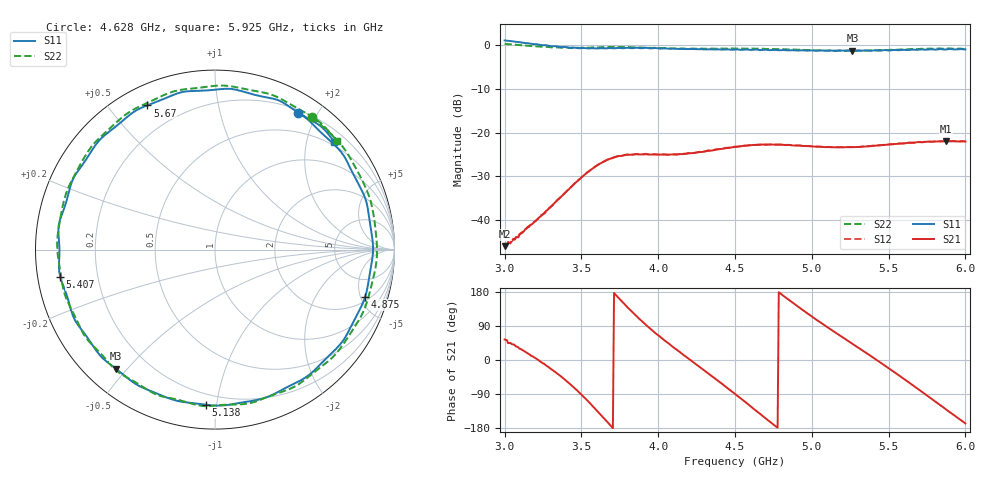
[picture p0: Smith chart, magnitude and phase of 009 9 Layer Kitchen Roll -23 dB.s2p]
!  04/11/2025  15:33:10
! Ref Plane: 0.000 mm
# MHZ S MA R  50
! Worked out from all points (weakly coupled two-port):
!   401 points, 3 GHz to 6 GHz, reference 50 ohm
!   highest |S21| = -22.00 dB at 5.872 GHz (marker M1); lowest = -46.0 dB at 3 GHz (marker M2)
!   lowest |S11| = -1.3 dB at 5.265 GHz (marker M3), VSWR 13.60, Z = 4.48 - j23.3 ohm
!   |S11| at or under -10 dB: nowhere
!   |S22| runs from -1.3 to 0.3 dB; largest |S21 - S12| = 0.0023
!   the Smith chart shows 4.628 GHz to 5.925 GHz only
!   S11 on the Smith chart (normalised r, x): 4.628 GHz: 0.24, +1.75; 4.875 GHz: 2.40, -5.49; 5.138 GHz: 0.14, -0.93; 5.407 GHz: 0.07, -0.09; 5.67 GHz: 0.08, +0.63; 5.925 GHz: 0.42, +2.54
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3000  1.134 -115.5  0.004996 54.1  0.004991 56.0  1.038 -119.1
3270  0.9997 176.6  0.01269 -14.1  0.01247 -11.4  0.9583 173.6
3390  0.9559 138.9  0.02013 -51.0  0.02016 -50.2  0.9414 135.3
3502.5  0.9284 96.3  0.03079 -92.3  0.0307 -91.6  0.9356 92.6
3607.5  0.9192 51.4  0.04263 -136.3  0.04271 -135.6  0.9427 48.3
3735  0.9306 -5.7  0.05337 166.9  0.05364 168.2  0.9537 -7.6
3862.5  0.9365 -58.1  0.05638 113.9  0.05669 115.5  0.9456 -59.2
4005  0.9178 -108.2  0.05589 63.7  0.0557 64.8  0.9252 -108.8
4245  0.8994 177.1  0.05878 -10.8  0.0589 -9.3  0.91 176.7
4500  0.8934 98.8  0.06853 -89.8  0.06902 -88.6  0.9148 95.9
4627.5  0.891 58.7  0.07197 -130.8  0.07201 -129.9  0.9123 53.8
4747.5  0.8826 21.2  0.07276 -169.5  0.07289 -168.3  0.9062 14.7
4875  0.8774 -17.5  0.0712 151.2  0.07122 152.4  0.8942 -24.9
5002.5  0.8727 -54.9  0.06924 114.3  0.06917 115.2  0.8802 -62.1
5137.5  0.8658 -93.3  0.06781 76.9  0.06789 77.9  0.8662 -99.5
5265  0.863 -129.7  0.06803 42.6  0.06826 43.5  0.8635 -133.8
5407.5  0.8757 -170.0  0.07067 4.0  0.0707 4.8  0.8707 -171.9
5505  0.8703 162.4  0.07289 -22.7  0.07332 -21.5  0.8852 161.4
5670  0.8873 115.2  0.07662 -70.2  0.07685 -68.8  0.9001 115.3
5872.5  0.8934 56.3  0.07944 -130.0  0.07996 -128.7  0.9131 56.7
5925  0.8958 42.1  0.07944 -145.1  0.07987 -143.9  0.9099 41.7
6000  0.8962 20.5  0.07882 -167.4  0.07912 -166.3  0.9061 19.7
